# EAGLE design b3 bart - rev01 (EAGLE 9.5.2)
COMPANY: ADAFRUIT INDUSTRIES; DRAWN: KTOWN; REV: B
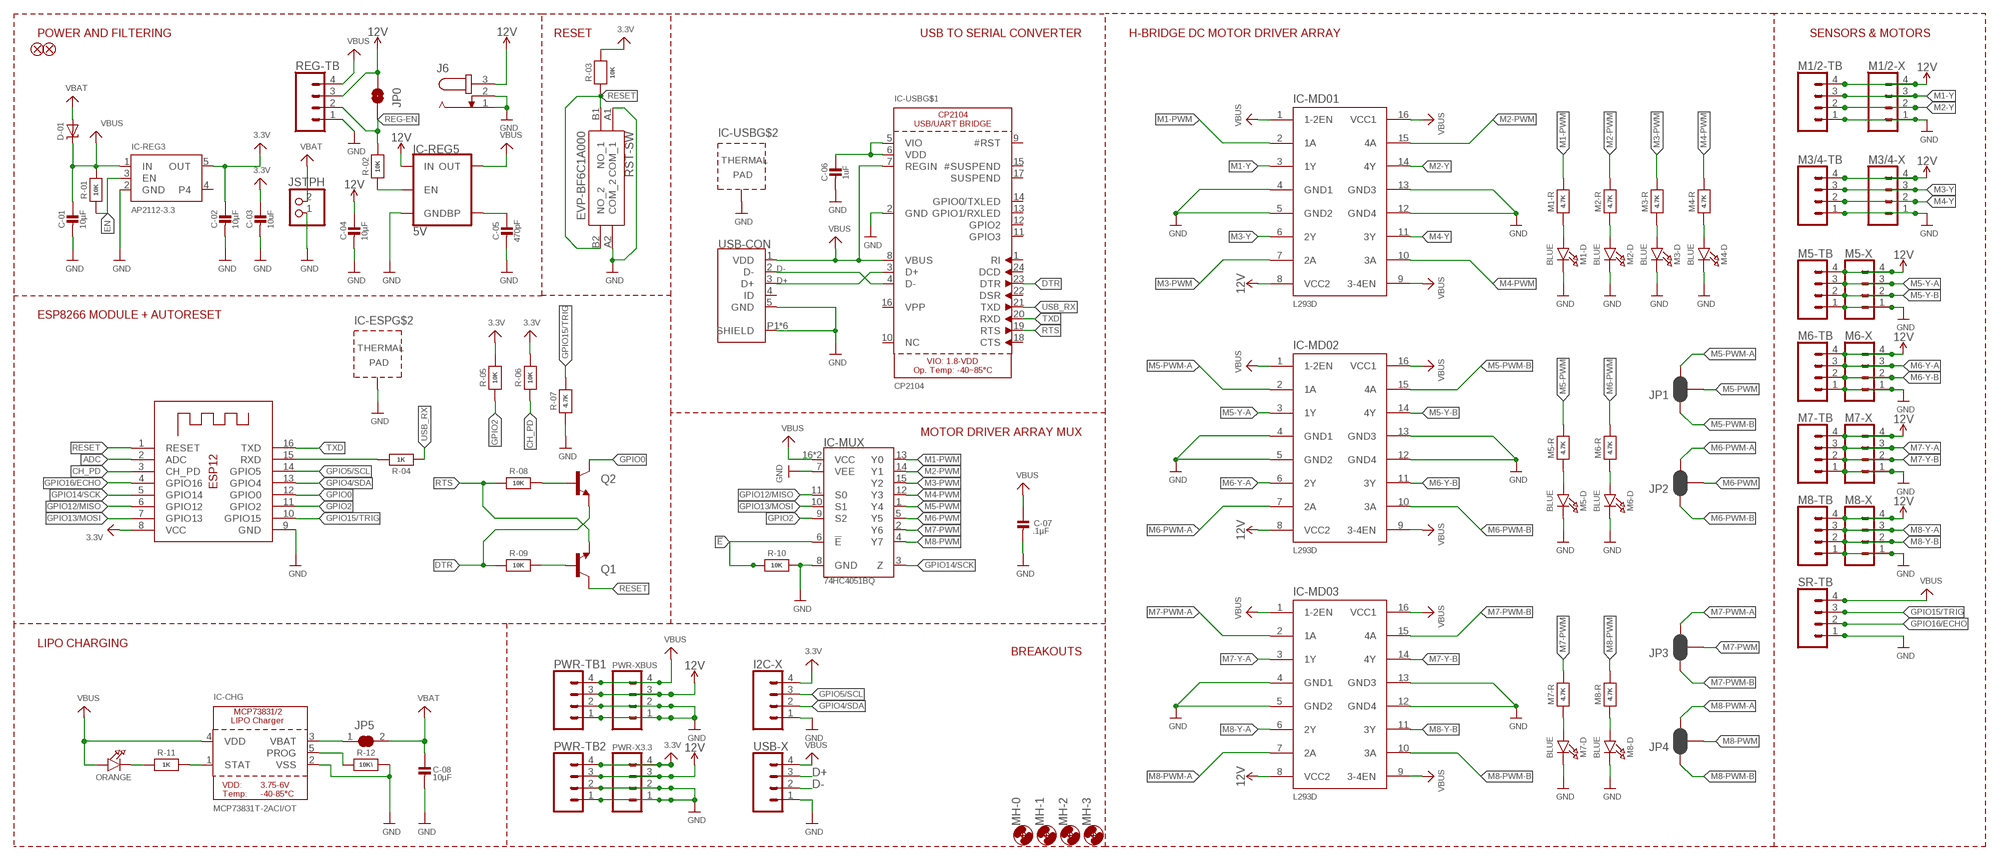
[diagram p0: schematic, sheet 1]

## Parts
C-01  10µF  CAP_CERAMIC0805-NOOUTLINE  [0805-NO]
C-02  10µF  CAP_CERAMIC0805-NOOUTLINE  [0805-NO]
C-03  10uF  CAP_CERAMIC0805-NOOUTLINE  [0805-NO]
C-04  10µF  CAP_CERAMIC0805-NOOUTLINE  [0805-NO]
C-05  470pF  CAP_CERAMIC0805-NOOUTLINE  [0805-NO]
C-06  1uF  CAP_CERAMIC0603_NO  [0603-NO@1]
C-07  .1µF  CAP_CERAMIC0805-NOOUTLINE  [0805-NO]
C-08  10µF  CAP_CERAMIC0805-NOOUTLINE  [0805-NO]
CHG-D  ORANGE  LED0805_NOOUTLINE  [CHIPLED_0805_NOOUTLINE]
D-01  MBR120  DIODE-SCHOTTKYSOD-123  [SOD-123]
FD1  FIDUCIAL1X2  [FIDUCIAL-1X2]
FD2  FIDUCIAL1X2  [FIDUCIAL-1X2]
I2C-X  CONN_04LONGPADS  [1X04_LONGPADS]
IC-CHG  MCP73831T-2ACI/OT  MCP73831/2  [SOT23-5]
IC-ESP  ESP-12  ESP-12S  [ESP-12S]
IC-MD01  L293D  [DIL16]
IC-MD02  L293D  [DIL16]
IC-MD03  L293D  [DIL16]
IC-MUX  74HC4051BQ  [DHVQFN-16-2.5X3.5MM]
IC-REG3  AP2112-3.3  VREG_SOT23-5  [SOT23-5]
IC-REG5  5V  V_REG_MIC52055V  [SOT23-5]
IC-USB  CP2104  [QFN24_4MM_SMSC]
J6  JACK-PLUG1  [SPC4078]
JP0  JUMPER-SMT_2_NO_SILK  [SMT-JUMPER_2_NO_SILK]
JP1  JUMPER-SMT_3_2-NC_PASTE_SILK  [SMT-JUMPER_3_2-NC_PASTE_SILK]
JP2  JUMPER-SMT_3_2-NC_PASTE_SILK  [SMT-JUMPER_3_2-NC_PASTE_SILK]
JP3  JUMPER-SMT_3_2-NC_PASTE_SILK  [SMT-JUMPER_3_2-NC_PASTE_SILK]
JP4  JUMPER-SMT_3_2-NC_PASTE_SILK  [SMT-JUMPER_3_2-NC_PASTE_SILK]
JP5  SOLDERJUMPER_CLOSED  [SOLDERJUMPER_CLOSEDWIRE]
M1-D  BLUE  LED0805_NOOUTLINE  [CHIPLED_0805_NOOUTLINE]
M1-R  4.7K  RESISTOR_0603_NOOUT  [0603-NO]
M1/2-TB  CONN_04SCREW  [SCREWTERMINAL-3.5MM-4]
M1/2-X  CONN_04LONGPADS  [1X04_LONGPADS]
M2-D  BLUE  LED0805_NOOUTLINE  [CHIPLED_0805_NOOUTLINE]
M2-R  4.7K  RESISTOR_0603_NOOUT  [0603-NO]
M3-D  BLUE  LED0805_NOOUTLINE  [CHIPLED_0805_NOOUTLINE]
M3-R  4.7K  RESISTOR_0603_NOOUT  [0603-NO]
M3/4-TB  CONN_04SCREW  [SCREWTERMINAL-3.5MM-4]
M3/4-X  CONN_04LONGPADS  [1X04_LONGPADS]
M4-D  BLUE  LED0805_NOOUTLINE  [CHIPLED_0805_NOOUTLINE]
M4-R  4.7K  RESISTOR_0603_NOOUT  [0603-NO]
M5-D  BLUE  LED0805_NOOUTLINE  [CHIPLED_0805_NOOUTLINE]
M5-R  4.7K  RESISTOR_0603_NOOUT  [0603-NO]
M5-TB  CONN_04SCREW  [SCREWTERMINAL-3.5MM-4]
M5-X  CONN_04LONGPADS  [1X04_LONGPADS]
M6-D  BLUE  LED0805_NOOUTLINE  [CHIPLED_0805_NOOUTLINE]
M6-R  4.7K  RESISTOR_0603_NOOUT  [0603-NO]
M6-TB  CONN_04SCREW  [SCREWTERMINAL-3.5MM-4]
M6-X  CONN_04LONGPADS  [1X04_LONGPADS]
M7-D  BLUE  LED0805_NOOUTLINE  [CHIPLED_0805_NOOUTLINE]
M7-R  4.7K  RESISTOR_0603_NOOUT  [0603-NO]
M7-TB  CONN_04SCREW  [SCREWTERMINAL-3.5MM-4]
M7-X  CONN_04LONGPADS  [1X04_LONGPADS]
M8-D  BLUE  LED0805_NOOUTLINE  [CHIPLED_0805_NOOUTLINE]
M8-R  4.7K  RESISTOR_0603_NOOUT  [0603-NO]
M8-TB  CONN_04SCREW  [SCREWTERMINAL-3.5MM-4]
M8-X  CONN_04LONGPADS  [1X04_LONGPADS]
MH-0  MOUNT-HOLE3.0  [3,0]
MH-1  MOUNT-HOLE3.0  [3,0]
MH-2  MOUNT-HOLE3.0  [3,0]
MH-3  MOUNT-HOLE3.0  [3,0]
PWR-TB1  CONN_04SCREW  [SCREWTERMINAL-3.5MM-4]
PWR-TB2  CONN_04SCREW  [SCREWTERMINAL-3.5MM-4]
PWR-X3.3  CONN_04LONGPADS  [1X04_LONGPADS]
PWR-XBUS  CONN_04LONGPADS  [1X04_LONGPADS]
Q1  mmbt2222  TRANSISTOR_NPNSOT23-3  [SOT23-3]
Q2  mmbt2222  TRANSISTOR_NPNSOT23-3  [SOT23-3]
R-01  10K  RESISTOR_0603_NOOUT  [0603-NO]
R-02  10K  RESISTOR_0603_NOOUT  [0603-NO]
R-03  10K  RESISTOR_0603_NOOUT  [0603-NO]
R-04  1K  RESISTOR_0603MP  [_0603MP]
R-05  10K  RESISTOR_0603_NOOUT  [0603-NO]
R-06  10K  RESISTOR_0603_NOOUT  [0603-NO]
R-07  4.7K  RESISTOR_0603_NOOUT  [0603-NO]
R-08  10K  RESISTOR_0603_NOOUT  [0603-NO]
R-09  10K  RESISTOR_0603_NOOUT  [0603-NO]
R-10  10K  RESISTOR_0603_NOOUT  [0603-NO]
R-11  1K  RESISTOR_0603_NOOUT  [0603-NO]
R-12  10K\  RESISTOR_0603_NOOUT  [0603-NO]
REG-TB  CONN_04SCREW  [SCREWTERMINAL-3.5MM-4]
RST-SW  EVP-BF6C1A000  [EVPBF6C1A000]
SR-TB  CONN_04SCREW  [SCREWTERMINAL-3.5MM-4]
USB-CON  10103592-0001LF  [AMPHENOL_10103592-0001LF]
USB-X  CONN_04LONGPADS  [1X04_LONGPADS]
X1  JSTPH  CON_JST_PH_2PIN  [JSTPH2]

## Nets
3.3V: C-02.1 C-03.1 I2C-X.4 IC-ESP.8(VCC) IC-REG3.5(OUT) PWR-TB2.4 PWR-X3.3.4 R-03.2 R-05.2 R-06.2
12V [power-motors]: C-04.1 IC-MD01.8(VCC2) IC-MD02.8(VCC2) IC-MD03.8(VCC2) IC-REG5.1(IN) J6.3 JP0.2 M1/2-TB.4 M1/2-X.4 M3/4-TB.4 M3/4-X.4 M5-TB.4 M5-X.4 M6-TB.4 M6-X.4 M7-TB.4 M7-X.4 M8-TB.4 M8-X.4 PWR-TB1.3 PWR-TB2.3 PWR-X3.3.3 PWR-XBUS.3 REG-TB.3
!E!: IC-MUX.6(!E!) R-10.1
ADC: IC-ESP.2(ADC)
CH_PD: IC-ESP.3(CH_PD) R-06.1
D+: IC-USB.3(D+) USB-CON.3(D+) USB-X.3
D-: IC-USB.4(D-) USB-CON.2(D-) USB-X.2
DTR: IC-USB.23(DTR) Q2.2(E) R-09.1
EN: IC-REG3.3(EN) R-01.1
GND: C-01.2 C-02.2 C-03.2 C-04.2 C-05.2 C-06.2 C-07.2 C-08.2 I2C-X.1 IC-CHG.2(VSS) IC-ESP.9(GND) IC-ESP.P$1(TP) IC-MD01.4(GND1) IC-MD01.5(GND2) IC-MD01.12(GND4) IC-MD01.13(GND3) IC-MD02.4(GND1) IC-MD02.5(GND2) IC-MD02.12(GND4) IC-MD02.13(GND3) IC-MD03.4(GND1) IC-MD03.5(GND2) IC-MD03.12(GND4) IC-MD03.13(GND3) IC-MUX.7(VEE) IC-MUX.8(GND) IC-REG3.2(GND) IC-REG5.2(GND) IC-USB.2(GND) IC-USB.THERM(TP) J6.1 J6.2 M1-D.C M1/2-TB.1 M1/2-X.1 M2-D.C M3-D.C M3/4-TB.1 M3/4-X.1 M4-D.C M5-D.C M5-TB.1 M5-X.1 M6-D.C M6-TB.1 M6-X.1 M7-D.C M7-TB.1 M7-X.1 M8-D.C M8-TB.1 M8-X.1 PWR-TB1.1 PWR-TB1.2 PWR-TB2.1 PWR-TB2.2 PWR-X3.3.1 PWR-X3.3.2 PWR-XBUS.1 PWR-XBUS.2 R-07.1 R-10.2 R-12.2 REG-TB.1 RST-SW.A1(COM_1) RST-SW.A2(COM_2) SR-TB.1 USB-CON.5(GND) USB-CON.P1(SHIELD) USB-CON.P2(SHIELD) USB-CON.P3(SHIELD) USB-CON.P4(SHIELD) USB-CON.P5(SHIELD) USB-CON.P6(SHIELD) USB-X.1 X1.1
GPIO0: IC-ESP.12(GPIO0) Q2.3(C)
GPIO2: IC-ESP.11(GPIO2) IC-MUX.9(S2) R-05.1
GPIO4/SDA: I2C-X.2 IC-ESP.13(GPIO4)
GPIO5/SCL: I2C-X.3 IC-ESP.14(GPIO5)
GPIO12/MISO: IC-ESP.6(GPIO12) IC-MUX.11(S0)
GPIO13/MOSI: IC-ESP.7(GPIO13) IC-MUX.10(S1)
GPIO14/SCK: IC-ESP.5(GPIO14) IC-MUX.3(Z)
GPIO15/TRIG: IC-ESP.10(GPIO15) R-07.2 SR-TB.3
GPIO16/ECHO: IC-ESP.4(GPIO16) SR-TB.2
M1-PWM: IC-MD01.2(1A) IC-MUX.13(Y0) M1-R.2
M1-Y [power-motors]: IC-MD01.3(1Y) M1/2-TB.3 M1/2-X.3
M2-PWM: IC-MD01.15(4A) IC-MUX.14(Y1) M2-R.2
M2-Y [power-motors]: IC-MD01.14(4Y) M1/2-TB.2 M1/2-X.2
M3-PWM: IC-MD01.7(2A) IC-MUX.15(Y2) M3-R.2
M3-Y [power-motors]: IC-MD01.6(2Y) M3/4-TB.3 M3/4-X.3
M4-PWM: IC-MD01.10(3A) IC-MUX.12(Y3) M4-R.2
M4-Y [power-motors]: IC-MD01.11(3Y) M3/4-TB.2 M3/4-X.2
M5-PWM: IC-MUX.1(Y4) JP1.2 M5-R.2
M5-PWM-A: IC-MD02.2(1A) JP1.3
M5-PWM-B: IC-MD02.15(4A) JP1.1
M5-Y-A [power-motors]: IC-MD02.3(1Y) M5-TB.3 M5-X.3
M5-Y-B [power-motors]: IC-MD02.14(4Y) M5-TB.2 M5-X.2
M6-PWM: IC-MUX.5(Y5) JP2.2 M6-R.2
M6-PWM-A: IC-MD02.7(2A) JP2.3
M6-PWM-B: IC-MD02.10(3A) JP2.1
M6-Y-A: IC-MD02.6(2Y) M6-TB.3 M6-X.3
M6-Y-B: IC-MD02.11(3Y) M6-TB.2 M6-X.2
M7-PWM: IC-MUX.2(Y6) JP3.2 M7-R.2
M7-PWM-A: IC-MD03.2(1A) JP3.3
M7-PWM-B: IC-MD03.15(4A) JP3.1
M7-Y-A: IC-MD03.3(1Y) M7-TB.3 M7-X.3
M7-Y-B: IC-MD03.14(4Y) M7-TB.2 M7-X.2
M8-PWM: IC-MUX.4(Y7) JP4.2 M8-R.2
M8-PWM-A: IC-MD03.7(2A) JP4.3
M8-PWM-B: IC-MD03.10(3A) JP4.1
M8-Y-A [power-motors]: IC-MD03.6(2Y) M8-TB.3 M8-X.3
M8-Y-B [power-motors]: IC-MD03.11(3Y) M8-TB.2 M8-X.2
N$1: CHG-D.C R-11.1
N$2: M5-D.A M5-R.1
N$3: IC-CHG.1(STAT) R-11.2
N$4: IC-CHG.5(PROG) R-12.1
N$5: M6-D.A M6-R.1
N$6: M1-D.A M1-R.1
N$7: IC-CHG.3(VBAT) JP5.1
N$8: C-06.1 IC-USB.5(VIO) IC-USB.6(VDD)
N$9: M2-D.A M2-R.1
N$10: IC-REG5.3(EN) R-02.1
N$11: M7-D.A M7-R.1
N$12: Q1.1(B) R-09.2
N$13: Q2.1(B) R-08.2
N$15: M8-D.A M8-R.1
N$18: M3-D.A M3-R.1
N$19: M4-D.A M4-R.1
N$21: C-05.1 IC-REG5.4(BP)
REG-EN: JP0.1 R-02.2 REG-TB.2
RESET: IC-ESP.1(RESET) Q1.3(C) R-03.1 RST-SW.B1(NO_1) RST-SW.B2(NO_2)
RTS: IC-USB.19(RTS) Q1.2(E) R-08.1
RXD: IC-ESP.15(RXD) R-04.2
TXD: IC-ESP.16(TXD) IC-USB.20(RXD)
USB_RX: IC-USB.21(TXD) R-04.1
VBAT: C-08.1 D-01.A JP5.2 X1.2
VBUS: C-01.1 C-07.1 CHG-D.A D-01.C IC-CHG.4(VDD) IC-MD01.1(1-2EN) IC-MD01.9(3-4EN) IC-MD01.16(VCC1) IC-MD02.1(1-2EN) IC-MD02.9(3-4EN) IC-MD02.16(VCC1) IC-MD03.1(1-2EN) IC-MD03.9(3-4EN) IC-MD03.16(VCC1) IC-MUX.16(VCC) IC-MUX.EP(VCC) IC-REG3.1(IN) IC-REG5.5(OUT) IC-USB.7(REGIN) IC-USB.8(VBUS) PWR-TB1.4 PWR-XBUS.4 R-01.2 REG-TB.4 SR-TB.4 USB-CON.1(VDD) USB-X.4
Unconnected: IC-REG3.4 IC-USB.1(RI) IC-USB.9(#RST) IC-USB.10(NC) IC-USB.11(GPIO3) IC-USB.12(GPIO2) IC-USB.13(GPIO1/RXLED) IC-USB.14(GPIO0/TXLED) IC-USB.15(#SUSPEND) IC-USB.16(VPP) IC-USB.17(SUSPEND) IC-USB.18(CTS) IC-USB.22(DSR) IC-USB.24(DCD) USB-CON.4(ID)

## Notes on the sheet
- POWER AND FILTERING | RESET | USB TO SERIAL CONVERTER | H-BRIDGE DC MOTOR DRIVER ARRAY | SENSORS & MOTORS
- ESP8266 MODULE + AUTORESET
- MOTOR DRIVER ARRAY MUX
- LIPO CHARGING | BREAKOUTS

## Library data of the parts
C-01-C-08 = microbuilder:CAP_CERAMIC: Ceramic Capacitors
CHG-D M1-D M2-D M3-D M4-D M5-D M6-D M7-D M8-D = microbuilder:LED: LED
D-01 = microbuilder:DIODE-SCHOTTKY
FD1 FD2 = SparkFun-Aesthetics:FIDUCIAL: Fiducial Alignment Points
I2C-X M1/2-X M3/4-X M5-X M6-X M7-X M8-X PWR-X3.3 PWR-XBUS USB-X = SparkFun-Connectors:CONN_04: Multi connection point. Often used as Generic Header-pin footprint for 0.1 inch spaced/style header connections On any of the 0.1 inch spaced packages, you can populate with these: Break Away Headers - Straight (PRT-00116) Break Away Male Headers - Right Angle (PRT-00553) Female Headers (PRT-00115)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; PROD_ID: CONN-09696
IC-CHG = microbuilder:MCP73831/2: MCP73831/2 LIPO Charger VDD: 3.75 - 6V Temp -40 - 85°C Programmable Charge Rate: 15-500mA NOTE: STAT is a tri-state logic output on the MCP73831 and an open-drain output on the MCP73832. SOT23-5 with 4.2V output and tri-state logic on STAT = MCP73831T-2ACI/OT
IC-ESP = microbuilder:ESP-12S
IC-MD01-IC-MD03 = st-microelectronics:L293D: PUSH-PULL 4 CHANNEL DRIVER; MPN: L293D; OC_FARNELL: 9589619; OC_NEWARK: 56P8249
IC-MUX = 8mux:74HC4051: NXP 74HC4051 8-Channel Analog Multiplexer/Demultiplexer The 74HC4051; 74HCT4051 is a single-pole octal-throw analog switch (SP8T) suitable for use in analog or digital 8:1 multiplexer/demultiplexer applications. The switch features three digital select inputs (S0, S1 and S2), eight independent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; PROD_ID: IC-13334
IC-REG3 = microbuilder:VREG_SOT23-5: SOT23-5 Fixed Voltage Regulators Part Current Out V Out V In V Dropout θJA (°C/W) TJ (°C) Digikey Part No. ADP121 150mA 3.3V 3.4-5.5V 0.09V @ 150mA -- -- ADP121-AUJZ33R7CT-ND ADP121 150mA 3.0V 3.1-5.5V 0.09V @ 150mA -- -- ADP121-AUJZ30R7CT-ND ADP122 300mA 3.3V 3.4-5.5V 0.085V @ 300mA -- --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
IC-REG5 = SparkFun-IC-Power:V_REG_MIC5205: V_REG MIC5205 Standard 3.3V, 5V, and Adjustable 150mA LDO voltage regulator in SOT-23 layout. Micrel part MIC5205. BP (by-pass) pin is used to lower output noise with 470pF cap, may be left open. On the adjustable version BP is used to set output.; PROD_ID: VREG-00823
IC-USB = microbuilder:CP2104: CP2104 - USB to UART Bridge VDD Output: 3.45V
J6 = con-jack:JACK-PLUG: DC POWER JACK Power Jack, DC, Right Angle, Through Hole, Rated 5A at 16VDC, PC Terminals Distributor: Farnell (www.Farnell.de) Drawing: 84N1161.pdf / 84N1162.pdf Manufacturer: SPC Technology (www.spctechnology.com) Type: SPC4077 / SPC 4078; OC_FARNELL: unknown; OC_NEWARK: unknown
JP0 = SparkFun-Jumpers:JUMPER-SMT_2_NO: Normally open jumper
JP1-JP4 = SparkFun-Jumpers:JUMPER-SMT_3_2-NC_PASTE: Normally closed solder jumper (2 of 2 connections) This jumper has an aperture in the stencil to allow solder paste to bridge both connections. Both connections are normally closed (NC). Wick off the solder to open the connection(s). Reapply solder to reclose the connection(s).
JP5 = microbuilder:SOLDERJUMPER_CLOSED: Solder Jumper - Closed
M1-R M2-R M3-R M4-R M5-R M6-R M7-R M8-R R-01-R-09 R-10-R-12 = microbuilder:RESISTOR: Resistors
M1/2-TB M3/4-TB M5-TB M6-TB M7-TB M8-TB PWR-TB1 PWR-TB2 REG-TB SR-TB = SparkFun-Connectors:CONN_04: Multi connection point. Often used as Generic Header-pin footprint for 0.1 inch spaced/style header connections On any of the 0.1 inch spaced packages, you can populate with these: Break Away Headers - Straight (PRT-00116) Break Away Male Headers - Right Angle (PRT-00553) Female Headers (PRT-00115)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; PROD_ID: 2xCONN-08399; SF_ID: 2xPRT-08084
MH-0 MH-1-MH-3 = holes:MOUNT-HOLE: MOUNTING HOLE with drill center marker
Q1 Q2 = SparkFun:TRANSISTOR_NPN: Transistor NPN BJT configuration in SOT23 package. MMBT2222 is the common NPN we use. Double check BCE configuration again layout.
RST-SW = SamacSys_Parts:EVP-BF6C1A000: Tactile Switches 6x6x3.5mm 3.5N 0.32mm Travel Source: Datasheet; DESCRIPTION: Tactile Switches 6x6x3.5mm 3.5N 0.32mm Travel; HEIGHT: 3.7mm; MANUFACTURER_NAME: Panasonic; MANUFACTURER_PART_NUMBER: EVP-BF6C1A000; MOUSER_PART_NUMBER: 667-EVP-BF6C1A000; MOUSER_PRICE-STOCK: https://www.mouser.com/Search/Refine.aspx?Keyword=667-EVP-BF6C1A000
USB-CON = 10103592-0001LF:10103592-0001LF: Conn Micro USB Type B RCP 5 POS 0.65mm Solder RA SMD 5 Terminal 1 Port T/R; DESCRIPTION: USB - micro B USB 2.0 Receptacle Connector 5 Position Surface Mount, Right Angle; Through Hole; DIGI-KEY_PART_NUMBER: 609-4048-1-ND; DIGI-KEY_PURCHASE_URL: https://www.digikey.com/product-detail/en/amphenol-icc-fci/10103592-0001LF/609-4048-1-ND/2350355?utm_source=snapeda&utm_medium=aggregator&utm_campaign=symbol; MF: Amphenol ICC; MP: 10103592-0001LF; PACKAGE: None
X1 = microbuilder:CON_JST_PH_2PIN: JST 2-Pin Right-Angle Connector

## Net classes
0 default: width 0.254 mm, drill 0.406 mm, clearance 0.203 mm
2 power-motors: width 0.457 mm, drill 0.406 mm, clearance 0.305 mm

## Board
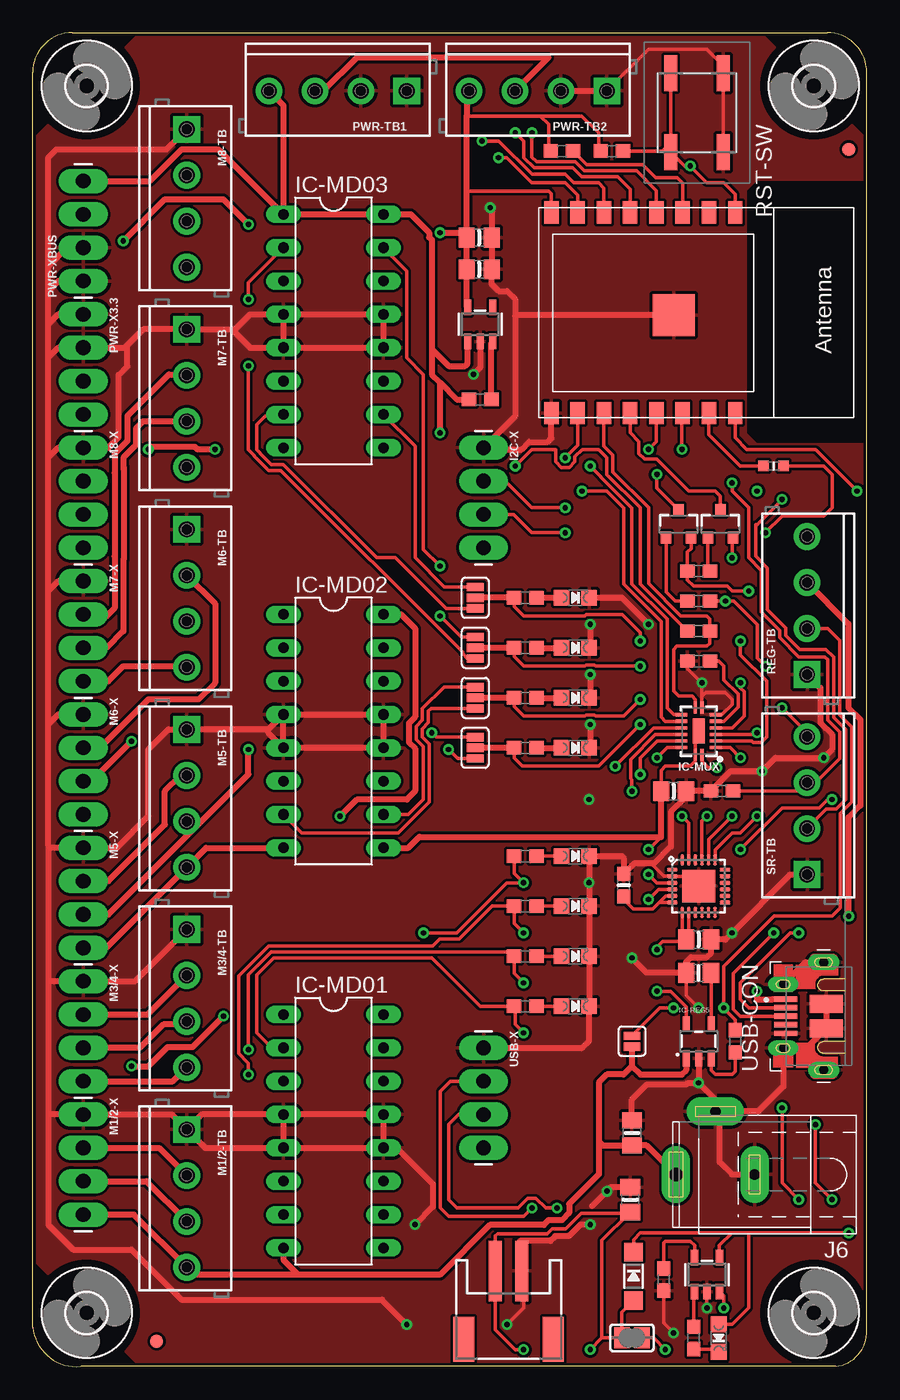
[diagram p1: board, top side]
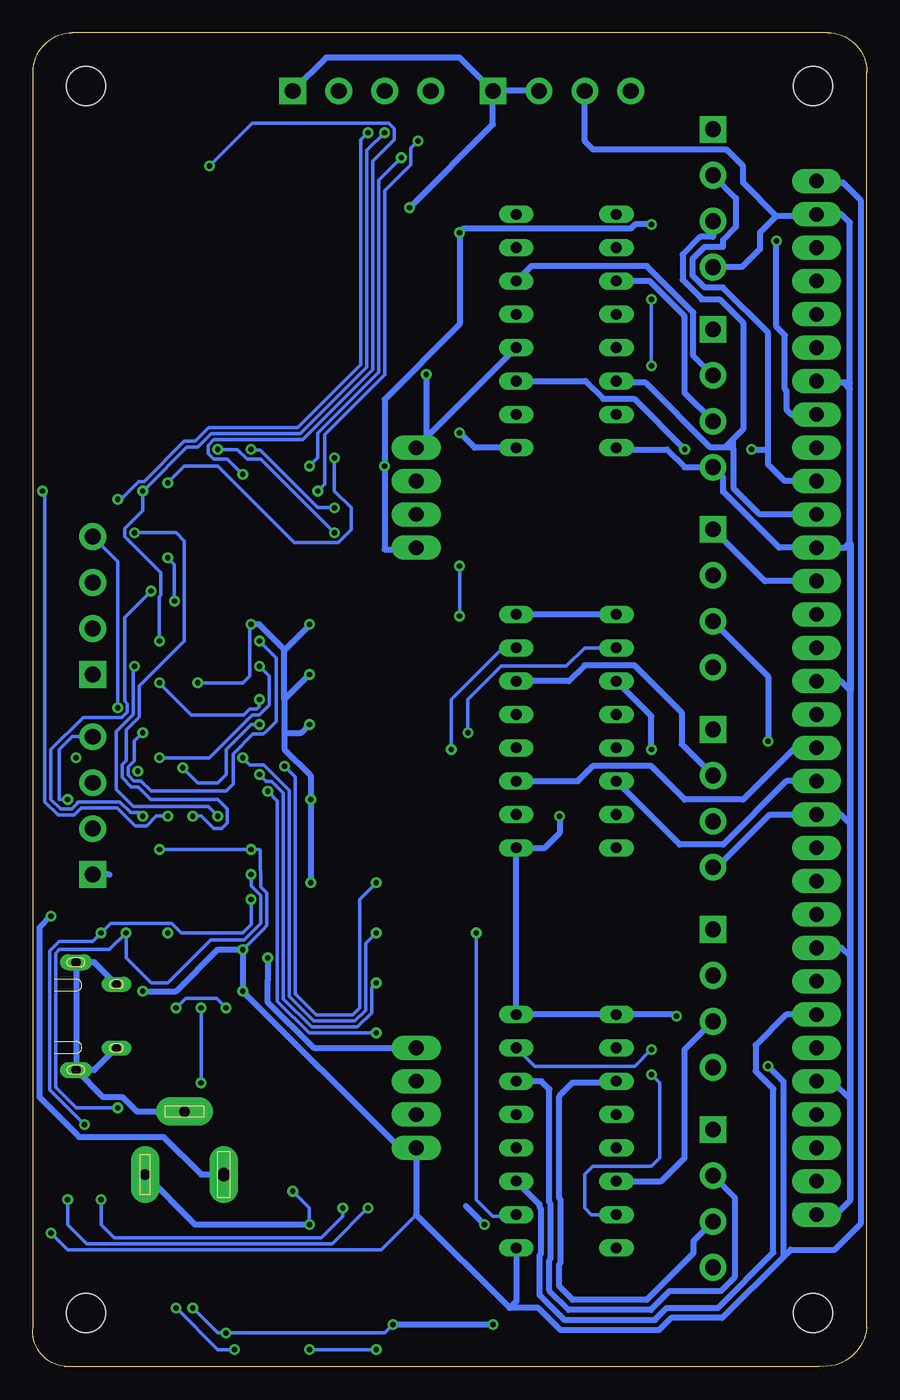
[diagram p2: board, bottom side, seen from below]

Size 63.52 x 101.62 mm. Coordinates in mm from the lower left corner, seen from the top.
Outline: 61.13,0.02 3.63,0.02 arc-90 0,3.02 0,98.62 arc-90 3,101.62 60.5,101.62 arc-90 63.5,98.62 63.5,3.02 arc-90 61.13,0.02
Copper layers (1*16): Top 0.035mm / dielectric 1.5mm / Bottom 0.035mm
Design rules "adafruit *": minimum track width 8mil, minimum drill 15.5mil, track to track 8mil, track to pad 8mil, pad to pad 8mil, via to via 8mil, smd to smd 8mil, copper to edge 10mil, drill to drill 8mil, minimum pad ring 10mil, minimum via ring 8mil, stop-mask expansion 2mil, vias tented up to drill 20mil, thermal gap 10mil
tKeepout: area 54.5,70.5 to 63.4,90.2; area 54.5,70.5 to 63.4,90.2
tRestrict: area 54.5,70.5 to 63.4,90.2

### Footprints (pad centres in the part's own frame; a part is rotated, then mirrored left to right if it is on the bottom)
0805-NO = smd 1.24 x 1.5: 1 -0.95,0; 2 0.95,0
0603-NO@1 = smd 1.075 x 1: 1 -0.85,0; 2 0.85,0
CHIPLED_0805_NOOUTLINE = smd 1.2 x 1.2: A 0,-1.05; C 0,1.05
SOD-123 = smd 1.4 x 1.4: A 1.85,0; C -1.85,0
FIDUCIAL-1X2 = smd 1 x 1: 1 0,0
1X04_LONGPADS = drill 1.118 pad 1.88 long: 1 0,0; 2 2.54,0; 3 5.08,0; 4 7.62,0
SOT23-5 = smd 0.55 x 1.2: 1 -0.95,-1.3; 2 0,-1.3; 3 0.95,-1.3; 4 0.95,1.3; 5 -0.95,1.3
ESP-12S = smd 1.7 x 1.1: 1 -7.65,5.77; 2 -7.65,3.77; 3 -7.65,1.77; 4 -7.65,-0.23; 5 -7.65,-2.23; 6 -7.65,-4.23; 7 -7.65,-6.23; 8 -7.65,-8.23; 9 7.65,-8.23; 10 7.65,-6.23; 11 7.65,-4.23; 12 7.65,-2.23; 13 7.65,-0.23; 14 7.65,1.77; 15 7.65,3.77; 16 7.65,5.77 | smd 3.2 x 3.2: P$1 0.2,1.1
DIL16 = drill 0.813 long: 1 -8.89,-3.81; 2 -6.35,-3.81; 3 -3.81,-3.81; 4 -1.27,-3.81; 5 1.27,-3.81; 6 3.81,-3.81; 7 6.35,-3.81; 8 8.89,-3.81; 9 8.89,3.81; 10 6.35,3.81; 11 3.81,3.81; 12 1.27,3.81; 13 -1.27,3.81; 14 -3.81,3.81; 15 -6.35,3.81; 16 -8.89,3.81
DHVQFN-16-2.5X3.5MM = smd 0.9 x 0.24: 1 -1.8,-0.25; 8 1.8,-0.25; 9 1.8,0.25; 16 -1.8,0.25 | smd 0.24 x 0.9: 2 -1.25,-1.3; 3 -0.75,-1.3; 4 -0.25,-1.3; 5 0.25,-1.3; 6 0.75,-1.3; 7 1.25,-1.3; 10 1.25,1.3; 11 0.75,1.3; 12 0.25,1.3; 13 -0.25,1.3; 14 -0.75,1.3; 15 -1.25,1.3 | smd 1.9 x 0.9: EP 0,0
QFN24_4MM_SMSC = smd 0.8 x 0.28: 1 -2,1.25; 2 -2,0.75; 3 -2,0.25; 4 -2,-0.25; 5 -2,-0.75; 6 -2,-1.25; 13 2,-1.25; 14 2,-0.75; 15 2,-0.25; 16 2,0.25; 17 2,0.75; 18 2,1.25 | smd 0.28 x 0.8: 7 -1.25,-2; 8 -0.75,-2; 9 -0.25,-2; 10 0.25,-2; 11 0.75,-2; 12 1.25,-2; 19 1.25,2; 20 0.75,2; 21 0.25,2; 22 -0.25,2; 23 -0.75,2; 24 -1.25,2 | smd 2.5 x 2.5: THERM 0,0
SPC4078 = drill 0.8 pad 2.184 long: 1 -3,0; 2 0,-4.8 | drill 1 pad 2.184 long: 3 3,0
SMT-JUMPER_2_NO_SILK = smd 0.635 x 1.27: 1 -0.406,0; 2 0.406,0
SMT-JUMPER_3_2-NC_PASTE_SILK = smd 0.635 x 1.27: 1 -0.813,0; 2 0,0; 3 0.813,0
SOLDERJUMPER_CLOSEDWIRE = smd 1.168 x 1.6: 1 -0.762,0; 2 0.762,0 | smd 0.635 x 0.203: WIRE 0,0
0603-NO = smd 1.1 x 1: 1 -0.85,0; 2 0.85,0
SCREWTERMINAL-3.5MM-4 = drill 1.2 pad 2.032 square: 1 0,0 | drill 1.2 pad 2.032: 2 3.5,0; 3 7,0; 4 10.5,0
3,0 = hole 3: 0,0
SOT23-3 = smd 0.8 x 0.9: 1 -0.95,-1; 2 0.95,-1; 3 0,1.1
_0603MP = smd 0.8 x 0.8: 1 -0.762,0; 2 0.762,0
EVPBF6C1A000 = smd 2.75 x 1: A1 3,-2; A2 -3,-2; B1 3,2; B2 -3,2
AMPHENOL_10103592-0001LF = smd 0.4 x 1.75: 1 1.3,2.875; 2 0.65,2.875; 3 0,2.875; 4 -0.65,2.875; 5 -1.3,2.875 | drill 0.65 pad 0.8 long: P1 -2.425,3.08; P2 2.425,3.08 | drill 0.7 pad 1.05 long: P3 -4.1,0; P6 4.1,0 | smd 1.375 x 2.5: P4 -0.938,-0.2; P5 0.938,-0.2
JSTPH2 = smd 1 x 4.6: 1 -1,-3.7; 2 1,-3.7 | smd 1.6 x 3.4: NC1 -3.4,1.5; NC2 3.4,1.5

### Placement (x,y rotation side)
C-01  50.7,32.54 0 top
C-02  33.99,83.6 0 top
C-03  33.99,86.01 0 top
C-04  45.62,17.81 90 top
C-05  50.7,30 180 top
C-06  44.99,36.68 90 top
C-07  48.8,43.85 0 top
C-08  45.5,12.73 90 top
CHG-D  52.23,2.19 180 top
D-01  45.75,6.89 270 top
FD1  62.13,92.74 0 top
FD2  9.43,1.94 0 top
I2C-X  34.32,70.01 270 top
IC-CHG  51.34,7.02 0 top
IC-ESP  47.72,80.29 270 top
IC-MD01  22.89,17.94 270 top
IC-MD02  22.89,48.42 270 top
IC-MD03  22.89,78.9 270 top
IC-MUX  50.7,48.42 90 top
IC-REG3  34.07,79.41 0 top
IC-REG5  50.7,24.8 0 top
IC-USB  50.7,36.61 0 top
J6  51.98,14.64 180 top
JP0  45.62,24.8 270 top
JP1  33.69,47.15 90 top
JP2  33.69,50.96 270 top
JP3  33.69,54.77 270 top
JP4  33.69,58.58 270 top
JP5  45.62,2.19 180 top
M1-D  41.31,27.46 270 top
M1-R  37.5,27.46 180 top
M1/2-TB  11.72,18.06 270 top
M1/2-X  3.84,19.21 270 top
M2-D  41.31,31.27 270 top
M2-R  37.5,31.27 180 top
M3-D  41.31,35.08 270 top
M3-R  37.5,35.08 180 top
M3/4-TB  11.72,33.3 270 top
M3/4-X  3.84,29.37 270 top
M4-D  41.31,38.89 270 top
M4-R  37.5,38.89 180 top
M5-D  41.31,47.15 270 top
M5-R  37.5,47.15 180 top
M5-TB  11.72,48.54 270 top
M5-X  3.84,39.53 270 top
M6-D  41.31,50.96 270 top
M6-R  37.5,50.96 180 top
M6-TB  11.72,63.78 270 top
M6-X  3.84,49.69 270 top
M7-D  41.31,54.77 270 top
M7-R  37.5,54.77 180 top
M7-TB  11.72,79.02 270 top
M7-X  3.84,59.85 270 top
M8-D  41.31,58.58 270 top
M8-R  37.5,58.58 180 top
M8-TB  11.72,94.26 270 top
M8-X  3.84,70.01 270 top
MH-0  4.1,97.57 0 top
MH-1  59.47,4.09 0 top
MH-2  4.1,4.09 0 top
MH-3  59.47,97.57 0 top
PWR-TB1  28.48,97.19 180 top
PWR-TB2  43.72,97.19 180 top
PWR-X3.3  3.84,80.17 270 top
PWR-XBUS  3.84,82.71 90 top
Q1  49.18,64.17 0 top
Q2  52.36,64.17 0 top
R-01  34.07,73.69 180 top
R-02  53.5,24.8 90 top
R-03  44.1,92.61 180 top
R-04  56.42,68.61 180 top
R-05  50.7,56.04 180 top
R-06  40.29,92.61 180 top
R-07  52.48,43.85 0 top
R-08  50.7,60.61 0 top
R-09  50.7,58.32 180 top
R-10  50.7,53.75 180 top
R-11  50.32,2.19 90 top
R-12  48.04,6.63 270 top
REG-TB  58.96,52.74 90 top
RST-SW  50.58,95.53 90 top
SR-TB  58.96,37.5 90 top
USB-CON  60.23,26.7 90 top
USB-X  34.32,24.29 270 top
X1  36.23,3.59 180 top

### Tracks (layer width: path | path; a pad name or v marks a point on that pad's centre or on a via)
3.3V  (via drill 0.41)
  Top 0.254: R-05.2 46.26,59.63 46.26,65.44 43.72,67.98 43.72,69.25 43.09,69.88 41.83,69.88 41.28,69.34 41.28,68.94 40.85,68.51 40.24,68.51 39.81,68.94 39.81,69.88 38.01,69.88 v36.73,68.61 | R-03.2 43.09,92.78 43.09,94.01 41.81,95.28 38.64,95.28 | IC-ESP.8 39.49,89.35 39.27,89.57 33.04,89.57 | 38.64,95.28 33.04,95.28 | R-06.2 39.27,92.78 39.27,94.65 38.64,95.28
  Top 0.457: IC-REG3.5 33.04,80.78 C-02.1 C-03.1 | v6.89,85.76 10.06,88.93 14.51,88.93 v16.42,87.03 | v31.02,86.39 32.66,86.39 C-03.1 | C-03.1 33.04,89.57 33.04,95.28 33.04,97.01 PWR-TB2.4
  Bottom 0.457: PWR-X3.3.4 5.75,72.55 6.13,72.93 6.13,74.35 6.25,74.48 6.25,78.58 6.89,79.21 v6.89,85.76 | v16.42,87.03 17.64,87.03 17.97,86.7 30.71,86.7 v31.02,86.39 31.02,79.41 36.73,73.69 v36.73,68.61 36.73,62.26 34.45,62.26 I2C-X.4
12V  (via drill 0.41)
  Top 0.457: J6.3 46.75,16.86 C-04.1 43.4,16.86 43.11,17.15 | IC-REG5.1 49.76,22.58 49.44,22.26 46.26,22.26 45.62,22.89 | 45.62,22.89 44.99,22.26 43.72,22.26 43.11,21.65 43.11,17.15 | 20.23,7.02 31.02,7.02 34.8,10.8 38.91,10.8 39.27,11.16 40.3,11.16 40.85,11.71 40.85,12.4 43.11,14.66 43.11,17.15 | 20.23,7.02 19.08,8.16 IC-MD01.8 | 20.23,7.02 12.26,7.02 M1/2-TB.4 7.69,11.59 M1/2-X.4 | M3/4-X.4 10.66,21.75 M3/4-TB.4 | M5-X.4 5.58,31.91 M5-TB.4 13.2,39.53 IC-MD02.8 | M7-X.4 5.75,52.23 6.89,53.37 11.63,53.37 M6-TB.4 | v62.13,34.32 62.13,41.86 63.02,42.74 63.02,49.29 62.11,50.2 62.11,56.59 REG-TB.3 | PWR-TB2.3 39.26,99.73 24.67,99.73 22.13,97.19 PWR-TB1.3 | JP0.2 45.62,22.89
  Bottom 0.457: 1.81,74.96 3.71,74.96 PWR-X3.3.3 | 6.89,87.66 3.97,87.66 PWR-XBUS.3 1.94,87.79 1.3,87.15 1.3,74.96 | 6.89,87.66 8.16,86.39 8.16,85.12 9.52,83.76 M8-TB.4 | 1.3,62.77 1.3,74.45 | 1.3,74.45 1.3,74.96 | 1.3,62.77 1.68,62.39 M8-X.4 6.69,62.39 10.96,66.65 10.96,67.77 M7-TB.4 13.88,68.52 15.23,69.88 18.96,69.88 IC-MD03.8 | 1.3,74.96 1.81,74.96 | 1.3,74.45 1.81,74.96 | J6.3 50.7,14.64 53.58,17.51 59.98,17.51 63.02,20.54 63.02,33.44 v62.13,34.32 | M5-X.4 1.94,31.91 1.25,31.22 | 1.25,12.73 1.25,20.35 | 1.25,20.35 1.25,31.22 | M1/2-X.4 2.39,11.59 1.25,12.73 | 1.25,20.35 2.64,21.75 M3/4-X.4 | 1.25,31.22 1.25,41.31 | 1.25,41.31 2.01,42.07 M6-X.4 7.4,42.07 11.42,38.04 M5-TB.4 | 1.25,41.31 1.25,51.47 | 1.25,51.47 2.01,52.23 M7-X.4 | 1.25,51.47 1.25,62.71 1.3,62.77 | 1.3,62.77 1.3,12.79 1.25,12.73 | 6.89,87.66 9.43,90.2 9.43,91.47 10.67,92.72 20.85,92.72 21.48,93.35 PWR-TB1.3
!E!
  Top 0.254: R-10.1 52.23,53.75 52.61,53.37 52.61,52.33 53.7,51.24 53.7,50.26 52.61,49.17 IC-MUX.6
CH_PD
  Top 0.254: IC-ESP.3 49.49,90.15 49.06,90.58 47.43,90.58 46.44,91.57 42.18,91.57 R-06.1
D+  (via drill 0.41)
  Top 0.254: IC-USB.3 48.17,36.86 48.16,36.86 47.53,36.86 v46.9,37.5 | USB-CON.3 53.88,26.7 53.35,27.23 53.35,29.98 v56.42,33.05 | USB-X.3 32.42,19.21 31.66,18.45 31.66,12.73 32.29,12.1 36.96,12.1 37.7,12.83 38.31,12.83 39.05,12.1 v39.91,12.1 | v57.05,19.72 57.05,14 v58.33,12.73
  Bottom 0.254: v46.9,37.5 46.9,36.63 46.16,35.9 46.16,33.79 46.44,33.51 46.44,33.5 47.42,32.52 49.97,32.52 53.25,29.24 54.52,29.24 56.42,31.15 v56.42,33.05 57.69,31.78 61.49,31.78 61.77,31.5 61.77,21.27 60.22,19.72 v57.05,19.72 | v58.33,12.73 58.33,10.83 57.33,9.83 41.54,9.83 39.91,11.46 v39.91,12.1
D-  (via drill 0.41)
  Top 0.254: IC-USB.4 47.66,36.36 v46.9,35.59 | USB-CON.2 57.34,27.34 54.52,27.34 53.88,27.97 53.88,29.24 57.69,33.05 v58.33,33.05 | USB-X.2 31.78,21.75 31.02,20.99 31.02,12.1 31.66,11.46 37.37,11.46 v38.01,12.1 | v59.59,18.45 59.59,14 v60.87,12.73
  Bottom 0.254: v46.9,35.59 46.9,33.69 47.53,33.05 52.2,33.05 52.94,33.79 57.59,33.79 v58.33,33.05 58.96,32.42 61.5,32.42 62.23,31.69 62.23,21.08 v59.59,18.45 | v60.87,12.73 60.87,10.83 59.42,9.38 40.72,9.38 v38.01,12.1
DTR  (via drill 0.41)
  Top 0.254: IC-USB.23 49.95,41.42 v49.44,41.94 | v55.79,53.37 55.15,54.01 55.15,56.55 53.37,58.32 v52.74,58.32 R-09.1 | v53.25,61.63 53.25,63.1 Q2.2
  Bottom 0.254: v49.44,41.94 50.17,42.68 55.89,42.68 57.18,43.97 57.18,48.38 55.86,49.7 55.86,53.29 v55.79,53.37 | v52.74,58.32 52.74,61.12 v53.25,61.63
EN
  Top 0.457: R-01.1 34.92,78.01 IC-REG3.3
GND  (via drill 0.41)
  Top 0.254: 51.98,32.54 C-01.2 | IC-USB.THERM 50.7,36.86 50.07,37.5 49.93,37.36 IC-USB.2 48.68,37.39 48.05,37.39 47.2,38.23 47.31,38.35 | C-05.2 49.76,28.3 50.7,27.35 v50.7,27.34 | IC-CHG.2 v51.34,4.48 | v48.8,2.57 48.04,3.33 R-12.2 | v36.1,3.21 37.37,4.48 37.37,7.14 X1.1 37.23,8.79 37.1,8.92 | 45.69,38.23 45.61,38.15 | IC-MUX.7 52.46,49.67 53.25,50.45 53.25,50.83 52.71,51.36 51.25,51.36 50.95,51.07 | IC-MUX.8 50.95,51.07 | 50.95,51.07 v50.95,52.1 49.86,53.2 R-10.2 | RST-SW.A2 RST-SW.A1 52.58,99.12 51.34,100.36 46.9,100.36 PWR-TB2.1
  Top 0.457: J6.2 55.24,19.44 57.15,21.35 USB-CON.P1 58.94,24.28 USB-CON.P4 USB-CON.P5 | J6.2 52.29,19.12 52.29,15.59 53.25,14.64 J6.1 | C-04.2 45.62,20.35 46.77,21.49 49.75,21.49 49.88,21.62 v50.7,21.62 | v50.7,21.62 51.98,20.35 J6.2 | IC-REG5.2 v50.7,21.62 | 51.98,32.54 52.74,32.54 v53.25,33.05 57.69,37.5 SR-TB.1 | C-01.2 51.66,31.5 51.34,31.18 50.11,31.18 49.76,30.83 C-05.2 46.77,30 v45.62,31.15 | M1/2-TB.1 10.57,19.21 M1/2-X.1 1.3,19.21 1.18,19.08 | M1/2-TB.1 13.11,16.67 IC-MD01.5 | IC-MD01.5 26.58,16.67 | 26.58,16.67 IC-MD01.12 27.72,16.67 30.46,13.92 30.46,12.17 v29.12,10.83 | M3/4-TB.1 7.78,29.37 M3/4-X.1 1.3,29.37 1.18,29.24 | 1.3,39.53 M5-X.1 6.38,39.53 8.79,41.94 8.79,47.02 10.32,48.54 M5-TB.1 17.94,48.54 | 1.3,39.53 1.18,39.4 1.18,29.24 | 1.18,29.24 1.18,19.08 | 1.18,19.08 1.18,10.83 3.08,8.92 7.53,8.92 11.33,5.11 26.58,5.11 v28.48,3.21 | C-08.2 44.04,13.68 v43.72,13.37 42.6,12.24 | 1.3,39.53 1.18,39.65 1.18,48.93 | 1.18,48.93 1.18,59.09 | 1.18,59.09 1.18,69.25 | 1.18,69.25 1.18,76.87 | 1.18,76.87 1.18,79.41 | 1.18,79.41 1.18,81.95 | 1.18,81.95 1.18,83.85 | 1.18,83.85 2.57,85.25 PWR-XBUS.2 | PWR-XBUS.1 1.94,82.71 1.18,81.95 | PWR-X3.3.1 1.94,80.17 1.18,79.41 | 1.18,76.87 1.94,77.63 PWR-X3.3.2 7.02,77.63 7.21,77.82 | 1.18,69.25 1.94,70.01 M8-X.1 5.75,70.01 6.53,70.79 6.53,75.54 7.21,76.21 7.21,77.82 | M7-X.1 1.94,59.85 1.18,59.09 | IC-MD03.4 IC-MD03.5 | 15.14,79.02 M7-TB.1 8.41,79.02 7.21,77.82 | 15.14,79.02 15.4,79.02 16.54,80.17 IC-MD03.4 | 15.14,79.02 16.54,77.63 IC-MD03.5 | IC-MD03.4 IC-MD03.13 IC-MD03.12 IC-MD03.5 | M6-X.1 1.94,49.69 1.18,48.93 | IC-MD01.4 IC-MD01.5 | 26.58,16.67 26.7,16.79 IC-MD01.13 IC-MD01.4
  Top 0.457: IC-MD01.4 12.86,19.21 M1/2-TB.1 | IC-MD02.4 IC-MD02.13 IC-MD02.12 IC-MD02.5 | IC-MD02.5 IC-MD02.4 | IC-MD02.4 17.94,48.54 | IC-MD02.5 17.94,48.29 17.94,48.54 | 1.18,83.85 1.18,92.11 1.81,92.74 10.19,92.74 M8-TB.1 | C-06.2 44.99,38.77 44.86,38.89 M4-D.C v42.36,36.86 M3-D.C M2-D.C M1-D.C 42.36,24.8 41.85,24.29 USB-X.1 | 45.69,38.23 C-06.2 | REG-TB.1 59.98,51.72 59.98,49.04 60.87,48.15 60.87,47.02 v60.23,46.39 56.55,46.39 v55.53,45.37 53.16,45.37 R-07.1 C-07.2 49.75,43.44 48.6,42.29 48.6,39.63 47.31,38.35 45.8,38.35 45.61,38.15 C-06.2 | M8-D.C 44.86,58.58 v46.9,56.55 | v42.45,52.74 42.45,51.05 M6-D.C | v42.45,48.93 42.45,47.24 M5-D.C | v42.45,56.55 42.45,54.86 M7-D.C | v34.83,88.3 34.94,88.18 C-03.2 C-02.2 34.94,82.47 35.47,81.95 36.1,81.95 36.73,81.31 36.73,80.04 | IC-REG3.2 34.07,76.1 v33.56,75.6 | IC-ESP.9 39.49,70.73 39.2,70.44 37.77,70.44 37.22,69.88 34.45,69.88 I2C-X.1 36.73,72.42 36.73,80.04 | PWR-TB2.2 PWR-TB2.1 | IC-ESP.P$1 36.79,80.09 36.73,80.04 | USB-CON.P2 58.83,30.8 USB-CON.P6 | 37.1,8.92 37.1,9.58 39.42,9.58 39.77,9.94 40.8,9.94 41.69,10.83 v42.45,10.83
  Bottom 0.254: v50.7,27.34 v50.7,21.62 | v51.34,4.48 49.44,2.57 v48.8,2.57 36.73,2.57 v36.1,3.21 | v42.45,10.83 42.45,12.1 v43.72,13.37 | v50.95,52.1 47.53,52.1 47,52.63 47,56.44 v46.9,56.55
  Bottom 0.457: v42.45,10.83 51.16,10.83 J6.1 | M7-X.1 7.78,59.85 M6-TB.1 | 30.53,12.24 v29.12,10.83 | v45.62,31.15 45.62,29.43 45.65,29.41 45.65,27.81 42.13,24.29 USB-X.1 | v42.36,36.86 v42.36,43.21 42.36,45.02 44.36,47.02 44.36,48.29 | 44.36,50.83 44.36,54.56 | 44.36,50.83 44.36,48.29 | 44.36,50.83 v42.45,52.74 | 44.36,48.29 43.09,48.29 v42.45,48.93 | 44.36,54.56 42.45,56.46 v42.45,56.55 | 44.36,54.56 44.36,54.64 46.26,56.55 v46.9,56.55 | PWR-TB1.2 PWR-TB1.1 | PWR-TB2.1 41.18,99.73 31.02,99.73 PWR-TB1.1 | v33.56,75.6 33.56,70.77 | 33.56,70.77 I2C-X.1 | IC-MD03.12 33.56,70.77 | 57.69,37.5 SR-TB.1 | USB-CON.P3 USB-CON.P6 58.83,30.8 USB-CON.P2 | USB-CON.P3 58.18,20.55 56.71,20.55 55.59,19.44 J6.2 | USB-CON.P1 58.83,22.6 USB-CON.P3 | v28.48,3.21 v36.1,3.21 | v34.83,88.3 28.48,94.65 PWR-TB1.1
  pour Top: 0.03,8.16 8.16,0.03 58.58,0.03 63.41,4.86 63.41,93.63 55.53,101.5 8.03,101.5 0.03,93.5
GPIO0
  Top 0.254: Q2.3 52.36,66.32 51.98,66.71 49.94,66.71 47.5,69.14 46.59,69.14 46.16,69.58 46.16,70.48 45.49,71.15 IC-ESP.12
GPIO2
  Top 0.254: IC-MUX.9 50.45,50.83 50.2,51.08 49.19,51.08 48.8,51.47 48.8,54.64 49.05,54.89 51.34,54.89 51.55,55.11 R-05.1 51.55,56.97 51.34,57.18 49.36,57.18 46.9,59.64 46.9,65.45 44.18,68.16 44.18,69.43 43.49,70.12 IC-ESP.11
GPIO4/SDA  (via drill 0.41)
  Top 0.254: IC-ESP.13 47.49,70.48 v46.9,69.88 | v40.55,65.44 38.01,65.44 35.97,67.47 I2C-X.2
  Bottom 0.254: v40.55,65.44 41.8,65.44 46.19,69.82 46.83,69.82 v46.9,69.88
GPIO5/SCL  (via drill 0.41)
  Top 0.254: I2C-X.3 36.61,64.93 38.01,63.53 v40.55,63.53 | v49.44,69.88 49.44,72.59 IC-ESP.14
  Bottom 0.254: v49.44,69.88 47.94,69.88 47.2,69.14 46.16,69.14 v40.55,63.53
GPIO12/MISO  (via drill 0.41)
  Top 0.254: IC-MUX.11 48.16,49.17 47.85,49.49 47.85,56.75 44.99,59.61 44.99,65.41 43.7,66.71 v41.81,66.71 | IC-ESP.6 43.49,89.79 43.09,90.2 41.19,90.2 40.56,90.84 38.02,90.84 35.48,93.38 v34.2,93.38
  Bottom 0.254: v41.81,66.71 41.28,67.24 41.28,71 36.71,75.57 36.71,89.59 34.73,91.57 34.73,92.84 v34.2,93.38
GPIO13/MOSI  (via drill 0.41)
  Top 0.254: IC-MUX.10 48.8,49.67 48.3,50.16 48.3,56.94 45.62,59.62 45.62,65.42 43.26,67.79 43.26,67.8 v42.45,68.61 | IC-ESP.7 41.49,89.26 40.55,90.2 38.01,90.2 36.1,92.11 v35.47,92.11
  Bottom 0.254: v42.45,68.61 41.81,69.25 41.81,71.12 37.17,75.76 37.17,90.4 v35.47,92.11
GPIO14/SCK  (via drill 0.41)
  Top 0.254: v53.88,55.28 53.88,54.23 55.89,52.23 55.89,47.99 55.45,47.55 54.84,47.55 54.73,47.67 IC-MUX.3 | IC-ESP.5 45.49,89.7 44.53,90.66 41.8,90.66 41.13,91.33 38.17,91.33 37.38,92.12 37.38,93.36 v36.73,94.01
  Bottom 0.254: v53.88,55.28 53.88,58.68 53.78,58.78 53.78,60.48 56.52,63.23 56.52,63.84 55.15,65.21 v55.15,66.71 54.87,66.98 54.86,66.98 51.79,70.06 50.95,70.06 49.93,71.07 43.15,71.07 38.08,76.14 38.08,92.66 v36.73,94.01
GPIO15/TRIG  (via drill 0.41)
  Top 0.254: R-07.2 58.31,43.85 SR-TB.3 59.61,44.5 61.44,46.33 61.44,48.36 60.54,49.27 60.54,53.86 60.31,54.08 58.33,54.08 56.88,55.53 56.88,56.1 55.47,57.5 55.47,60.67 54.52,61.63 54.52,65.44 54.2,65.75 53.25,66.71 v53.25,67.34 | IC-ESP.10 41.49,70.19 v40.55,69.25
  Bottom 0.254: v40.55,69.25 40.55,66.71 39.27,65.44 39.27,63.76 40.24,62.79 43.62,62.79 49.44,68.61 51.98,68.61 v53.25,67.34
GPIO16/ECHO  (via drill 0.41)
  Top 0.254: SR-TB.2 60.44,42.47 61.17,42.47 61.9,43.2 61.9,48.55 60.99,49.46 60.99,54.05 60.4,54.64 58.41,54.64 57.33,55.72 57.33,56.29 55.93,57.69 55.93,60.86 55.05,61.74 55.05,64.17 55.15,64.17 v57.05,66.07 | IC-ESP.4 47.49,89.61 45.98,91.11 41.99,91.11 41.33,91.78 38.36,91.78 38.01,92.14 v38.01,94.01
  Bottom 0.254: v57.05,66.07 56.83,66.07 55.45,67.44 55.05,67.44 51.98,70.52 51.13,70.52 50.12,71.53 43.34,71.53 38.54,76.33 38.54,93.47 v38.01,94.01
M1-PWM  (via drill 0.41)
  Top 0.254: IC-MD01.2 18.19,24.29 17.05,25.43 17.05,29.84 18.36,31.15 30.39,31.15 34.07,27.46 M1-R.2 36.73,27.37 36.73,26.07 v37.37,25.43 | v45.62,43.85 45.62,44.71 45.52,44.81 45.52,46.27 47.42,48.17 IC-MUX.13
  Bottom 0.254: v37.37,25.43 42.45,25.43 42.47,25.41 44.89,27.83 44.89,43.11 v45.62,43.85
M1-Y
  Top 0.457: M1/2-X.3 8.65,14.13 M1/2-TB.3
  Bottom 0.457: IC-MD01.3 20.1,21.75 20.2,21.65 22.4,21.65 23.43,20.62 23.43,12.81 23.32,12.71 23.32,7.92 23.43,7.82 23.43,6.11 22.4,5.09 16.78,5.09 13.21,8.65 13.21,9.57 M1/2-TB.3
M2-PWM  (via drill 0.41)
  Top 0.254: v16.42,24.16 16.42,29.85 18.17,31.6 36.32,31.6 M2-R.2 36.65,29.96 v37.37,29.24 | v46.26,45.12 46.26,46.36 47.56,47.67 IC-MUX.14
  Bottom 0.254: v16.42,24.16 17.69,22.89 25.3,22.89 IC-MD01.15 | v37.37,29.24 37.73,28.88 37.73,26.96 38.8,25.89 42.3,25.89 44.43,28.02 44.43,43.69 45.32,44.58 45.73,44.58 v46.26,45.12
M2-Y
  Top 0.457: M1/2-X.2 9.61,16.67 M1/2-TB.2
  Bottom 0.457: M1/2-TB.2 10.06,12.91 10.06,6.82 11.14,5.75 15.04,5.75 16.46,4.32 22.72,4.32 24.19,5.79 24.19,8.14 24.09,8.24 24.09,12.4 24.19,12.5 24.19,21.14 24.8,21.75 IC-MD01.14
M3-PWM  (via drill 0.41)
  Top 0.254: v16.42,22.26 16.42,23.12 15.68,23.86 15.68,29.76 17.98,32.06 30.46,32.06 30.99,32.59 32.48,32.59 34.97,35.08 M3-R.2 36.65,33.77 v37.37,33.05 | v47.53,46.39 48.31,47.17 IC-MUX.15
  Bottom 0.254: v16.42,22.26 15.78,21.62 15.78,15.91 16.42,15.27 20.86,15.27 21.5,14.64 21.5,12.1 20.99,11.59 IC-MD01.7 | v37.37,33.05 38.18,32.24 38.18,27.15 38.98,26.34 42.11,26.34 43.97,28.21 43.97,43.88 45.94,45.85 47,45.85 v47.53,46.39
M3-Y
  Top 0.457: M3/4-X.3 8.16,24.29 9.94,26.07 11.48,26.07 M3/4-TB.3
  Bottom 0.457: IC-MD01.6 15.65,14.13 13.88,15.91 13.88,24.16 11.73,26.3 M3/4-TB.3
M4-PWM  (via drill 0.41)
  Top 0.254: v44.36,45.75 47.27,48.67 IC-MUX.12 | M4-R.2 36.65,37.58 v37.37,36.86 36.1,36.86 32.29,33.05 v29.75,33.05
  Bottom 0.254: v29.75,33.05 29.75,12.73 28.48,11.46 26.83,11.46 IC-MD01.10 | v37.37,36.86 38.64,35.59 38.64,27.34 39.17,26.8 41.92,26.8 43.52,28.4 43.52,44.91 v44.36,45.75
M4-Y
  Top 0.457: M3/4-X.2 8.74,26.83 M3/4-TB.2
  Bottom 0.457: M3/4-X.2 6.13,26.83 8.46,24.49 8.46,22.5 7.11,21.15 7.11,8.7 11.33,4.48 15.23,4.48 16.14,3.56 23.04,3.56 24.95,5.48 24.95,8.45 24.85,8.55 24.85,12.08 24.95,12.18 24.95,12.37 IC-MD01.11
M5-PWM  (via drill 0.41)
  Top 0.254: IC-MUX.1 50.95,46.14 51.47,45.62 v52.1,45.62 | M5-R.2 36.65,46.39 37.28,45.75 43.09,45.75 v46.26,48.93
  Top 0.457: M5-R.2 JP1.2
  Bottom 0.254: v52.1,45.62 50.96,44.48 49.44,44.48 48.8,45.12 48.8,47.01 46.88,48.93 v46.26,48.93
M5-PWM-A  (via drill 0.41)
  Top 0.254: JP1.3 30.71,47.96 v30.39,48.29
  Bottom 0.254: IC-MD02.2 21.5,54.77 22.89,53.37 27.85,53.37 30.39,50.83 v30.39,48.29
M5-PWM-B  (via drill 0.41)
  Top 0.254: JP1.1 32.34,46.33 v31.66,47.02
  Bottom 0.254: v31.66,47.02 31.66,50.83 27.72,54.77 IC-MD02.15
M5-Y-A  (via drill 0.41)
  Top 0.457: M5-X.3 5.75,34.45 11.33,40.04 11.72,40.42 | 11.72,40.42 M5-TB.3 | 11.72,40.42 16.42,45.12 v16.42,47.02
  Bottom 0.457: v16.42,47.02 16.42,49.56 IC-MD02.3
M5-Y-B
  Top 0.457: M5-X.2 5.75,36.99 10.06,41.31 10.06,43.85 11.26,45.04 M5-TB.2
  Bottom 0.457: M5-TB.2 14.1,47.43 14.1,49.84 17.69,53.42 21.5,53.42 22.69,52.23 IC-MD02.14
M6-PWM  (via drill 0.41)
  Top 0.254: IC-MUX.5 53.25,48.67 54.16,49.58 54.16,51.43 53.88,51.71 v53.88,52.1 | M6-R.2 36.65,50.28 37.37,49.56 42.04,49.56 42.15,49.66 42.76,49.66 42.86,49.56 44.99,49.56 v46.26,50.83
  Top 0.457: M6-R.2 JP2.2
  Bottom 0.254: v53.88,52.1 51.44,49.66 47.44,49.66 46.98,50.12 46.45,50.12 46.26,50.31 v46.26,50.83
M6-PWM-A
  Top 0.254: JP2.3 30.33,50.14 30.13,49.94 30.13,49.08 29.65,48.6 29.65,47.99 30.21,47.43 30.21,43.03 27.85,40.67 20.48,40.67 IC-MD02.7
M6-PWM-B
  Top 0.254: JP2.1 31.31,51.77 29.67,50.13 29.67,49.27 29.19,48.78 29.19,47.8 29.75,47.24 29.75,43.22 28.6,42.07 IC-MD02.10
M6-Y-A  (via drill 0.41)
  Top 0.457: v7.53,47.66 4.48,44.61 M6-X.3
  Bottom 0.457: M6-X.3 6.13,44.61 10.95,39.78 14.26,39.78 IC-MD02.6 | M6-TB.3 7.53,52.59 v7.53,47.66
M6-Y-B
  Top 0.457: M6-TB.2 13.88,58.13 13.88,52.1 12.6,50.83 8.79,50.83 5.11,47.15 M6-X.2
  Bottom 0.457: IC-MD02.11 22,44.61 20.86,45.75 16.42,45.75 13.88,43.21 9.43,43.21 5.49,47.15 M6-X.2
M7-PWM  (via drill 0.41)
  Top 0.254: IC-MUX.2 53.1,47.17 v53.88,46.39 | M7-R.2 36.65,54.09 37.37,53.37 42.04,53.37 42.15,53.47 42.76,53.47 42.86,53.37 v46.26,53.37
  Top 0.457: M7-R.2 JP3.2
  Bottom 0.254: v53.88,46.39 50.07,46.39 46.79,49.66 46.26,49.66 45.52,50.4 45.52,52.63 v46.26,53.37
M7-PWM-A  (via drill 0.41)
  Top 0.254: v16.42,81.31 16.42,82.58 IC-MD03.2 | v16.42,76.23 16.42,69.87 16.87,69.41 16.87,69.37 17.97,68.26 18.89,68.26 32.72,54.44 32.72,54.31 33.08,53.95 JP3.3
  Bottom 0.254: v16.42,76.23 v16.42,81.31
M7-PWM-B  (via drill 0.41)
  Top 0.254: JP3.1 32.62,55.58 v31.02,57.18 | IC-MD03.15 28.48,83.47 28.48,76.87 29.75,75.6 29.75,62.26 v31.02,60.99
  Bottom 0.254: v31.02,60.99 v31.02,57.18
M7-Y-A
  Top 0.457: M7-X.3 5.62,54.77 6.89,56.04 6.89,61.48 6.92,61.5 6.92,68.59 6.89,68.61 | M7-TB.3 8.4,72.02 7.86,71.48 7.86,70.21 6.89,69.25 6.89,68.61 | 6.89,68.61 6.89,68.38 6.92,68.35
  Bottom 0.457: IC-MD03.3 16.54,82.71 13.88,80.04 13.88,74.18 M7-TB.3
M7-Y-B
  Top 0.457: M7-X.2 3.97,57.18 5.62,57.18 6.23,57.79 6.23,61.75 6.25,61.78 6.25,68.08 6.23,68.1 6.23,69.55 7.2,70.52 7.2,72.42 10.37,75.6 11.64,75.6 M7-TB.2
  Bottom 0.457: IC-MD03.14 25.56,83.85 16.75,83.85 13.21,80.31 13.21,77.02 M7-TB.2
M8-PWM  (via drill 0.41)
  Top 0.254: v55.15,48.29 55.03,48.17 IC-MUX.4 | v46.26,55.28 46.26,55.91 44.89,57.28 42.15,57.28 42.04,57.18 37.37,57.18 36.65,57.9 M8-R.2
  Top 0.457: M8-R.2 JP4.2
  Bottom 0.254: v55.15,48.29 55.79,47.66 55.79,46.16 56.27,45.67 56.27,45.06 55.84,44.63 55.3,44.63 54.52,43.85 48.8,43.85 48.27,44.38 48.27,46.69 46.77,48.19 45.95,48.19 45.74,48.4 45.52,48.62 44.99,49.15 44.99,54.01 v46.26,55.28
M8-PWM-A
  Top 0.254: IC-MD03.7 18.96,72.42 17.69,72.42 17.05,71.79 17.05,69.88 17.33,69.6 17.33,69.56 18.16,68.72 19.08,68.72 26.18,61.63 27.62,61.63 31.48,57.76 JP4.3
M8-PWM-B
  Top 0.254: JP4.1 31.35,59.39 29.12,61.63 29.12,70.13 IC-MD03.10
M8-Y-A
  Bottom 0.457: IC-MD03.6 18.96,74.96 16.86,74.96 11.97,70.07 10.7,70.07 | M8-TB.3 11.72,86.08 12.67,86.08 14.03,84.72 14.03,82.81 12.6,81.38 12.6,81.31 11.22,81.31 9.43,79.52 9.43,71.41 10.17,70.67 | M8-X.3 8.15,64.93 10.17,66.94 10.17,69.88 | 10.17,69.88 10.17,70.67 | 10.17,69.88 10.36,70.07 10.7,70.07 | 10.17,70.67 10.7,70.14 10.7,70.07
M8-Y-B  (via drill 0.41)
  Top 0.457: v13.88,69.88 12.55,69.88 12.36,70.07 8.99,70.07 v8.79,69.88
  Bottom 0.457: IC-MD03.11 21.43,75.09 20.08,73.74 17.74,73.74 v13.88,69.88 | M8-TB.2 9.97,89.02 9.97,86.82 10.95,85.84 10.95,85.31 12.36,85.31 13.26,84.41 13.26,83.12 12.36,82.22 10.97,82.22 7.53,78.77 7.53,69.88 | v8.79,69.88 7.53,69.88 | 7.53,69.88 7.53,68.74 6.25,67.47 M8-X.2
N$1
  Top 0.254: R-11.1 52.03,1.34 CHG-D.C
N$2
  Top 0.457: M5-R.1 M5-D.A
N$3
  Top 0.254: R-11.2 50.32,5.65 IC-CHG.1
N$4
  Top 0.254: IC-CHG.5 50.39,9.24 50.07,9.56 48.16,9.56 48.04,9.43 R-12.1
N$5
  Top 0.457: M6-R.1 M6-D.A
N$6
  Top 0.254: M1-R.1 M1-D.A
N$7  (via drill 0.41)
  Top 0.254: IC-CHG.3 52.61,5.4 v52.61,4.48 | v48.16,1.3 47.28,2.19 JP5.1
  Bottom 0.254: v52.61,4.48 49.44,1.3 v48.16,1.3
N$8
  Top 0.254: IC-USB.6 47.7,35.36 | 47.7,35.36 47.2,34.85 45.73,34.85 44.99,35.59 C-06.1 | IC-USB.5 48.2,35.86 47.7,35.36
N$9
  Top 0.254: M2-R.1 40.42,31.27
  Top 0.457: M2-D.A 40.42,31.27
N$10
  Top 0.254: IC-REG5.3 51.66,22.58 51.98,22.26 53.25,22.26 53.5,22.51 R-02.1
N$11
  Top 0.457: M7-R.1 M7-D.A
N$12
  Top 0.254: Q1.1 48.23,59.02 48.93,58.32 R-09.2
N$13
  Top 0.254: Q2.1 51.41,60.76 R-08.2
N$15
  Top 0.457: M8-R.1 M8-D.A
N$18
  Top 0.254: M3-R.1 M3-D.A
N$19
  Top 0.254: M4-R.1 M4-D.A
N$21
  Top 0.254: C-05.1 IC-REG5.4
REG-EN  (via drill 0.41)
  Top 0.254: JP0.1 47.76,27.34 v48.8,27.34 | REG-TB.2 60.54,56.24 61.45,55.33 61.45,49.65 62.36,48.74 62.36,43.01 61.48,42.13 61.48,34.93 60.89,34.35 56.45,34.35 52.61,30.51 v52.61,27.34 52.89,27.06 52.89,27.04 53.5,26.43 R-02.2
  Bottom 0.254: v52.61,27.34 51.87,28.07 49.64,28.07 49.62,28.05 49.51,28.05 v48.8,27.34
RESET  (via drill 0.41)
  Top 0.254: Q1.3 47.53,66.92 v47.53,67.98 | RST-SW.B1 48.58,93.25 | 48.58,93.25 RST-SW.B2 49.64,91.47 v50.07,91.47 51.34,90.2 52.61,90.2 53.49,89.32 IC-ESP.1 | R-03.1 47.94,92.61 48.58,93.25
  Bottom 0.254: v47.53,67.98 48.7,69.14 49.74,69.14 50.17,69.58 50.17,70.19 49.74,70.62 42.96,70.62 37.63,75.95 37.63,91.85 36,93.48 36,94.32 36.43,94.75 46.79,94.75 v50.07,91.47
RTS  (via drill 0.41)
  Top 0.254: IC-USB.19 51.95,39.38 53.25,40.67 53.88,40.67 v55.15,41.94 | Q1.2 50.13,62.32 49.86,62.05 R-08.1 49.86,59.94 50.32,59.47 52.86,59.47 53.25,59.09 v54.52,59.09
  Bottom 0.254: v55.15,41.94 55.43,42.22 56.08,42.22 56.89,43.03 60.06,43.03 60.13,42.97 60.13,42.91 60.56,42.47 61.41,42.47 62.13,43.2 62.13,47.02 59.7,49.46 56.75,49.46 56.32,49.89 56.32,50.5 56.52,50.7 56.52,57.08 v54.52,59.09
RXD
  Top 0.254: IC-ESP.15 51.49,71 53.88,68.61 R-04.2
TXD  (via drill 0.41)
  Top 0.254: IC-USB.20 51.45,40.15 v53.25,41.94 | IC-ESP.16 53.49,70.76 54.37,69.88 59.61,69.88 61.32,68.16 61.32,68.15 v62.77,66.71
  Bottom 0.254: v53.25,41.94 54.11,41.94 54.84,41.2 55.71,41.2 57.08,42.58 59.81,42.58 60.37,42.02 61.6,42.02 62.59,43.01 62.59,66.53 v62.77,66.71
USB_RX  (via drill 0.41)
  Top 0.254: IC-USB.21 50.95,41.56 v51.34,41.94 | R-04.1 60.23,68.61 60.87,67.98 60.87,65.44 60.23,64.8 57.05,64.8 v55.79,63.53
  Bottom 0.254: v51.34,41.94 50.7,41.94 49.75,40.99 49.12,40.99 48.7,41.41 48.7,42.47 49.44,43.21 54.53,43.21 55.49,44.18 56.02,44.18 56.73,44.88 56.73,45.86 56.42,46.17 56.42,48.5 55.4,49.51 55.4,51.85 51.98,55.28 51.98,62.9 52.61,63.53 v55.79,63.53
VBAT  (via drill 0.41)
  Top 0.254: D-01.A 44.86,4.15 JP5.2 43.34,2.19 | v37.37,1.3 36.73,1.3 35.23,2.81 X1.2 35.23,9.95 35.41,10.14 39.19,10.14 39.54,10.5 40.57,10.5 41.76,11.68 45.4,11.68 | v42.45,1.3 43.34,2.19 | 45.4,11.68 43.34,9.62 43.34,2.19 | 45.4,11.68 C-08.1
  Bottom 0.254: v37.37,1.3 v42.45,1.3
VBUS  (via drill 0.41)
  Top 0.254: IC-USB.8 49.95,32.74 C-01.1 | IC-USB.7 49.45,32.84 C-01.1 | C-01.1 49.63,32.42 47.96,32.42 47.43,31.88 v47.53,31.78 | CHG-D.A 53.28,3.24 54.52,4.48 54.52,10.19 | IC-CHG.4 52.29,9.24 53.25,10.19 | v62.13,10.19 54.52,10.19 | v46.9,39.4 47.85,40.35 29.43,40.35 | D-01.C 45.75,9.68 46.26,10.19 53.25,10.19 | 53.25,10.19 54.52,10.19 | IC-MUX.EP 50.45,48.17 IC-MUX.16 50.45,46.14 50.07,45.75 48.16,45.75 47.85,45.44 C-07.1 | v53.88,39.4 57.05,42.58 59.89,42.58 60.53,43.21 v60.87,43.21 | v57.05,50.2 58.96,48.29 SR-TB.4 | IC-REG5.5 49.76,27.42 48.57,28.61 v47.53,28.61
  Top 0.457: IC-MD03.1 IC-MD03.16 28.79,87.79 30.18,86.39 30.18,86.04 30.39,85.84 30.39,77.5 | v14.51,26.7 12.16,24.35 10.26,24.35 8.79,22.89 v7.53,22.89 | v23.4,41.94 24.67,43.21 28.48,43.21 29.12,43.85 29.12,47.08 28.63,47.56 28.63,49.02 29.12,49.5 29.12,56.25 28.05,57.31 IC-MD02.16 | IC-MD02.9 28.61,39.53 29.43,40.35 29.44,40.36 47.85,40.36 | 47.85,40.35 47.85,40.36 | 47.85,40.36 C-07.1 | PWR-TB1.4 19.08,96.08 IC-MD03.1 | PWR-XBUS.4 8.92,90.33 11.33,92.74 14.13,92.74 IC-MD03.1 | 30.39,77.5 30.39,75.6 31.02,74.96 | 31.02,74.96 32.29,73.69 R-01.2 | 30.39,77.5 31.66,76.23 32.93,76.23 33.12,76.42 IC-REG3.1 | v31.02,71.15 31.02,74.96 | USB-CON.1 57.34,27.98 56.3,27.98 56.29,27.97 55.15,27.97 v55.15,28.61
  Bottom 0.254: v53.88,39.4 v46.9,39.4 46.26,39.4 46.18,39.32 46.18,37.83 46.16,37.8 46.16,36.54 45.7,36.08 45.7,33.6 45.98,33.32 45.98,33.31 47.23,32.06 47.25,32.06 v47.53,31.78 | v60.87,43.21 61.5,43.21 61.5,47.01 60.51,48 SR-TB.4 | REG-TB.4 57.05,61.33 v57.05,50.2 | 34.32,11.59 36.99,8.92 60.87,8.92 v62.13,10.19
  Bottom 0.457: PWR-XBUS.4 3.71,90.2 1.81,90.2 0.48,88.87 0.48,10.88 2.44,8.92 5.81,8.92 6.35,8.38 | IC-MD01.9 26.7,4.98 27.21,4.48 | 6.35,8.38 11.02,3.71 14.91,3.71 15.83,2.8 23.35,2.8 25.03,4.48 27.21,4.48 | 6.35,8.38 6.35,21.72 v7.53,22.89 | v14.51,26.7 14.64,26.83 IC-MD01.1 IC-MD01.16 IC-MD02.9 24.54,39.53 23.4,40.67 v23.4,41.94 | IC-MD02.1 IC-MD02.16 | IC-MD03.9 29.88,70.01 v31.02,71.15 | v55.15,28.61 52.61,28.61 49.44,31.78 v47.53,31.78 v47.53,28.61 35.59,16.67 USB-X.4 34.32,11.59 27.21,4.48

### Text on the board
tSilk: Edward Daniel Nichols - BART / University of Central Florida SPG2020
